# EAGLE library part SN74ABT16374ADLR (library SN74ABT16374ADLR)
16-Bit Edge-Triggered D-Type Fflip-Flops With 3-State Outputs Source: Datasheet
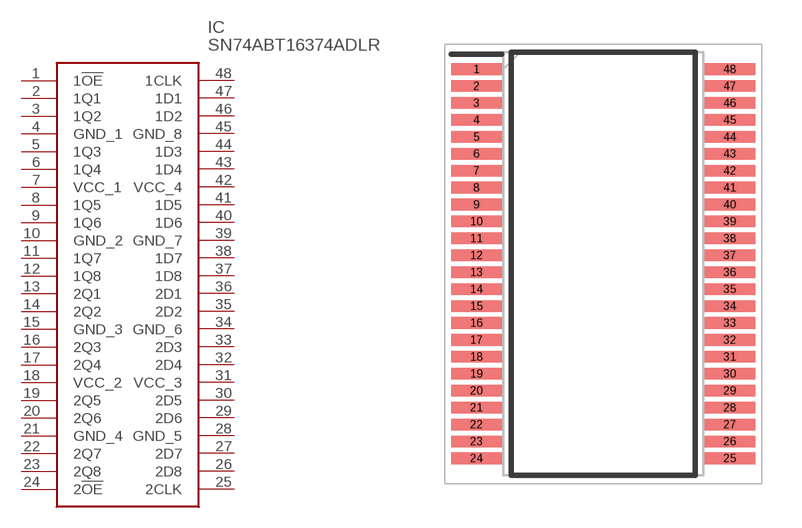
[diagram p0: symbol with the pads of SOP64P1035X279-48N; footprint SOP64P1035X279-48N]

Designator prefix IC

## SN74ABT16374ADLR (Description: 16-Bit Edge-Triggered D-Type Fflip-Flops With 3-State Outputs; Height: 2.79mm; Manufacturer_Name: Texas Instruments; Manufacturer_Part_Number: SN74ABT16374ADLR; Mouser_Part_Number: 595-SN74ABT16374ADLR; Mouser_Price-Stock: https://www.mouser.com/Search/Refine.aspx?Keyword=595-SN74ABT16374ADLR)  [SOP64P1035X279-48N]
1  1!OE
2  1Q1
3  1Q2
4  GND_1
5  1Q3
6  1Q4
7  VCC_1
8  1Q5
9  1Q6
10  GND_2
11  1Q7
12  1Q8
13  2Q1
14  2Q2
15  GND_3
16  2Q3
17  2Q4
18  VCC_2
19  2Q5
20  2Q6
21  GND_4
22  2Q7
23  2Q8
24  2!OE
25  2CLK
26  2D8
27  2D7
28  GND_5
29  2D6
30  2D5
31  VCC_3
32  2D4
33  2D3
34  GND_6
35  2D2
36  2D1
37  1D8
38  1D7
39  GND_7
40  1D6
41  1D5
42  VCC_4
43  1D4
44  1D3
45  GND_8
46  1D2
47  1D1
48  1CLK

## Footprint SOP64P1035X279-48N (pad centres in mm)
DL (R-PDSO-G48)
smd 1.9 x 0.435: 1 -4.75,7.302; 2 -4.75,6.668; 3 -4.75,6.032; 4 -4.75,5.398; 5 -4.75,4.762; 6 -4.75,4.128; 7 -4.75,3.492; 8 -4.75,2.858; 9 -4.75,2.222; 10 -4.75,1.588; 11 -4.75,0.952; 12 -4.75,0.318; 13 -4.75,-0.318; 14 -4.75,-0.952; 15 -4.75,-1.588; 16 -4.75,-2.222; 17 -4.75,-2.858; 18 -4.75,-3.492; 19 -4.75,-4.128; 20 -4.75,-4.762; 21 -4.75,-5.398; 22 -4.75,-6.032; 23 -4.75,-6.668; 24 -4.75,-7.302; 25 4.75,-7.302; 26 4.75,-6.668; 27 4.75,-6.032; 28 4.75,-5.398; 29 4.75,-4.762; 30 4.75,-4.128; 31 4.75,-3.492; 32 4.75,-2.858; 33 4.75,-2.222; 34 4.75,-1.588; 35 4.75,-0.952; 36 4.75,-0.318; 37 4.75,0.318; 38 4.75,0.952; 39 4.75,1.588; 40 4.75,2.222; 41 4.75,2.858; 42 4.75,3.492; 43 4.75,4.128; 44 4.75,4.762; 45 4.75,5.398; 46 4.75,6.032; 47 4.75,6.668; 48 4.75,7.302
